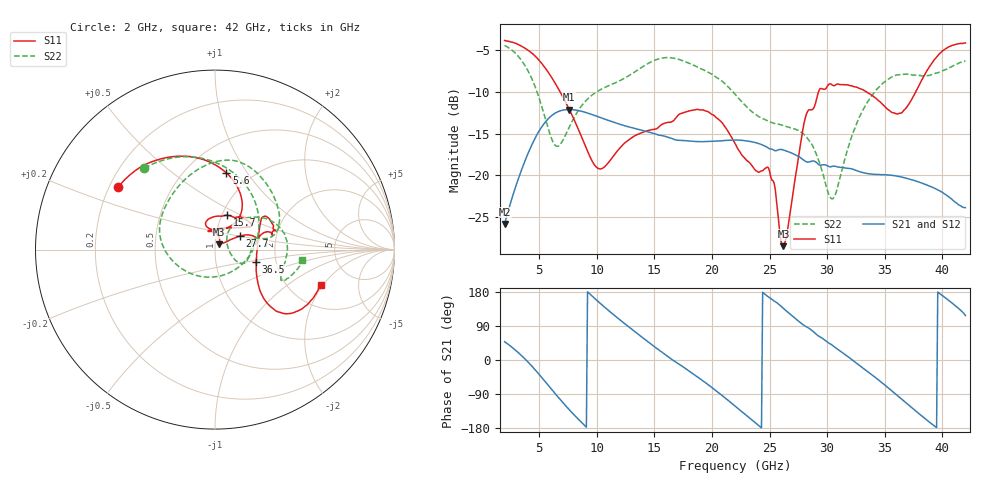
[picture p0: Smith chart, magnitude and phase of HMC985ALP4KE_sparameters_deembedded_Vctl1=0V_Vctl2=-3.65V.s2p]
!s2p File: Measurements: S11, S21, S12, S22
# GHz S dB R 50.0
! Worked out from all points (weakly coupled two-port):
!   401 points, 2 GHz to 42 GHz, reference 50 ohm
!   highest |S21| = -12.11 dB at 7.6 GHz (marker M1); lowest = -25.8 dB at 2 GHz (marker M2)
!   lowest |S11| = -28.5 dB at 26.2 GHz (marker M3), VSWR 1.08, Z = 52.3 + j3.12 ohm
!   |S11| at or under -10 dB: 6.818 GHz to 29.25 GHz (22.43 GHz wide, 124 % of centre); 33.42 GHz to 37.69 GHz (4.271 GHz wide, 12 % of centre)
!   |S22| runs from -22.8 to -4.4 dB; largest |S21 - S12| = 0.00031
!   S11 on the Smith chart (normalised r, x): 2 GHz: 0.24, +0.28; 5.6 GHz: 0.77, +0.81; 15.7 GHz: 1.06, +0.42; 27.7 GHz: 1.30, +0.20; 36.5 GHz: 1.57, -0.23; 42 GHz: 2.95, -1.89
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2  -3.85 146.9  -25.81 48.3  -25.81 48.3  -4.44 130.9
3.6  -4.64 120.0  -18.86 7.8  -18.86 7.8  -6.50 86.1
4.6  -5.66 101.2  -15.66 -24.1  -15.66 -24.0  -9.21 49.8
5.6  -7.29 81.6  -13.50 -59.8  -13.50 -59.8  -13.51 -0.6
6.5  -9.22 66.3  -12.46 -92.6  -12.45 -92.7  -16.50 -68.4
7.6  -12.05 54.4  -12.11 -130.8  -12.11 -130.8  -14.25 -138.4
8.7  -15.45 54.7  -12.33 -165.4  -12.33 -165.4  -11.63 -172.6
10.4  -19.20 90.3  -13.11 146.7  -13.10 146.8  -9.67 160.1
15.4  -14.19 75.6  -15.18 26.4  -15.18 26.4  -6.05 85.3
15.7  -13.85 70.3  -15.24 19.7  -15.25 19.7  -5.95 81.5
19.4  -12.26 33.2  -15.95 -59.1  -15.95 -59.1  -7.46 34.8
22  -16.16 51.4  -15.75 -121.4  -15.76 -121.4  -10.27 12.2
24.9  -19.07 104.5  -16.74 166.4  -16.73 166.4  -13.50 12.2
26.2  -28.45 52.0  -16.95 136.2  -16.96 136.2  -14.04 -4.0
27.7  -16.14 28.7  -17.88 98.0  -17.89 97.9  -14.78 -23.3
28.7  -12.12 12.7  -18.27 77.4  -18.27 77.4  -16.34 -29.0
30.5  -9.22 18.3  -18.89 37.8  -18.89 37.8  -22.78 18.5
32.9  -9.63 34.0  -19.58 -16.7  -19.58 -16.7  -12.73 47.7
35.4  -12.22 11.7  -19.95 -76.0  -19.95 -76.0  -8.40 19.2
36.5  -12.47 -16.6  -20.20 -104.1  -20.20 -104.1  -7.88 6.0
39.5  -5.85 -43.6  -21.65 -178.4  -21.64 -178.4  -7.74 -24.7
42  -4.15 -18.5  -23.84 117.2  -23.84 117.3  -6.26 -6.8
